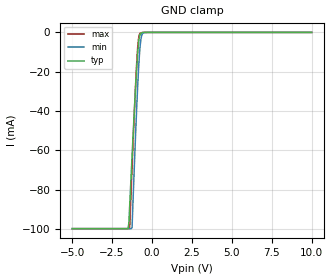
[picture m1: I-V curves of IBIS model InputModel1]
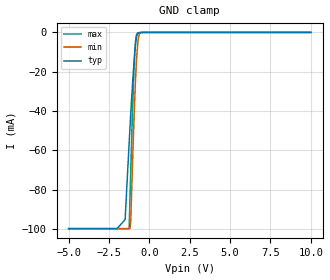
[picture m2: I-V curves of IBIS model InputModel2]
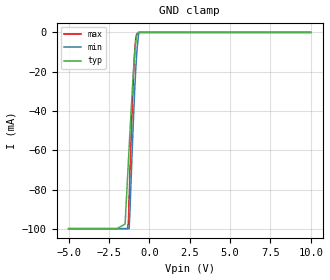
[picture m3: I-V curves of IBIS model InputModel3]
[IBIS Ver]   2.1
[File name]   e_002bl5.ibs   | e_= TSOP, f002bl= abbr chip name, 5= 5V Vcc
[File Rev]   2.00
[Date]   16-February-96
[Source]   File generated from lab measurements at Intel Corporation
[Notes]   Rev 2.00 All data was replaced by actual measurements
   performed in a lab.
[Disclaimer] INTEL DEVELOPER'S SOFTWARE LICENSE AGREEMENT
| BY USING THIS SOFTWARE, YOU ARE AGREEING TO BE BOUND
| BY THE TERMS OFTHIS AGREEMENT.  DO NOT USE THE SOFTWARE
| UNTIL YOU HAVE CAREFULLY READAND AGREED TO THE FOLLOWING
| TERMS AND CONDITIONS.  IF YOU DO NOT AGREETO THE TERMS
| OF THIS AGREEMENT, PROMPTLY RETURN THE SOFTWARE PACKAGE
| ANDANY ACCOMPANYING ITEMS.
| IF YOU USE THIS SOFTWARE, YOU WILL BE BOUND BY THE TERMS
| OF THIS AGREEMENT
| LICENSE: Intel Corporation ("Intel") grants you the non-exclusive right
| to use the enclosed software program ("Software").  You will not use,
| copy, modify, rent, sell or transfer the Software or any portion
| thereof, except as provided in this Agreement.
| System OEM Developers may:
| 1.   Copy the Software for support, backup or archival purposes;
| 2.   Install, use, or distribute Intel owned Software in object code
|   only;
| 3.   Modify and/or use Software source code that Intel directly makes
|   available to you as an OEM Developer;
| 4.   Install, use, modify, distribute, and/or make or have made
|   derivatives ("Derivatives") of Intel owned Software under the
|   terms and conditions in this Agreement, ONLY if you are a System
|   OEM Developer and NOT an end-user.
| RESTRICTIONS:
| YOU WILL NOT:
| 1.   Copy the Software, in whole or in part, except as provided for
|   in this Agreement;
| 2.   Decompile or reverse engineer any Software provided in object
|   code format;
| 3.   Distribute any Software or Derivative code to any end-users,
|   unless approved by Intel in a prior writing.
| TRANSFER: You may transfer the Software to another OEM
| Developer if thereceiving party agrees to the terms of this
| Agreement at the sole risk of any receiving party.
| OWNERSHIP AND COPYRIGHT OF SOFTWARE:
| Title to the Software and all copies thereof remain with Intel
| or its vendors.  The Software iscopyrighted and is protected by
| United States and international copyright laws.  You will not
| remove the copyright notice from the Software.  You agree to
| prevent any unauthorized copying of the Software.
| DERIVATIVE WORK: OEM Developers that make or have made
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[Copyright]   Copyright 1996, Intel Corporation, All Rights Reserved
[Component]   E28F002BL   | 40-lead TSOP package, 28F002BL
[Manufacturer]  Intel   | Boot Block (tm)
|   | operating in 5V Vcc range
[Package]
| The following values apply for the Alloy-42 leadframe.
|Variable   typ   min   max
R_pkg   135m   126m   144m
L_pkg   3.95nH   3.62nH   4.28nH
C_pkg   0.39pF   0.38pF   0.40pF
|***********************Pin Definition********************************
[Pin]   signal_name   model_name   R_pin   L_pin   C_pin
  1   A16   InputModel2
  2   A15   InputModel1
  3   A14   InputModel1
  4   A13   InputModel1
  5   A12   InputModel1
  6   A11   InputModel1
  7   A9   InputModel1
  8   A8   InputModel1
  9   WE#   InputModel5
 10   RP#   InputModel3
 11   VPP   POWER
 12   DU   InputModel6
 13   NC   InputModel1
 14   A7   InputModel1
 15   A6   InputModel1
 16   A5   InputModel1
 17   A4   InputModel1
 18   A3   InputModel1
 19   A2   InputModel1
 20   A1   InputModel1
 21   A0   InputModel2
 22   CE#   InputModel2
 23   GND   GND
 24   OE#   InputModel4
 25   DQ0   InputOutput
 26   DQ1   InputOutput
 27   DQ2   InputOutput
 28   DQ3   InputOutput
 29   NC   InputModel2
 30   VCC   POWER
 31   VCC   POWER
 32   DQ4   InputOutput
 33   DQ5   InputOutput
 34   DQ6   InputOutput
 35   DQ7   InputOutput
 36   A10   InputModel1
 37   NC   InputModel6
 38   NC   InputModel6
 39   GND   GND
 40   A17   InputModel1
|***********************Input Model 6******************************
[Model]   InputModel6
Model_type   Input
|   Model for  DU & NC pins, excluding Pin #13.
Vinl = 0.8V
Vinh = 2.0V
|Variable   Typ   Min   Max
C_comp   5.61p   NA   7.6p
[Voltage Range]   5.0V   4.5V   5.5V
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| Models and submodels in the file (7): InputModel1 (Input), InputModel2 (Input), InputModel3 (Input), InputModel4 (Input), InputModel5 (Input), InputModel6 (Input), InputOutput (I/O)
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|*********************Input Model 1************************************
[Model]   InputModel1
Model_type   Input
|   Model for A[15:1] A[17] & NC (pin 13).
Vinl = 0.8V
Vinh = 2.0V
|Variable   Typ   Min   Max
C_comp   5.61p   NA   7.6p
[Voltage Range]   5.0V   4.5V   5.5V
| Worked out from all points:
|   GND clamp passes 1 mA (typ) near -0.75 V on its own axis
[GND_clamp]
|Voltage  I(typ)   I(min)   I(max)
-5V       -99.84mA   -99.85mA   -99.85mA
-1.5V     -99.84mA   -99.85mA   -99.85mA
-1.45V    -97.1mA    -99.85mA   -99.85mA
-1.4V     -88.66mA   -99.85mA   -99.85mA
-1.25V    -63.24mA   -99.36mA   -69.05mA
-1.05V    -31.09mA   -56.35mA   -30.63mA
-950mV    -16.83mA   -36.7mA    -14.35mA
-850mV    -5.99mA    -19.86mA   -3.6mA
-750mV    -1.015mA   -7.435mA   -471.4uA
-650mV    -202.7uA   -1.654mA   -140.8uA
-500mV    -27.26uA   -101.4uA   -12.27uA
10V       0A         0A         0A
[Power_clamp]
| Input buffer circuits of this product do not intrinsically
| require a [Power_clamp] definition.  This zero current
| [Power_clamp] table is provided for the compatibility with
| some IBIS parsers.
|Voltage  I(typ)   I(min)   I(max)
-5V       0A         0A         0A
0V        0A         0A         0A
5V        0A         0A         0A
10V       0A         0A         0A
|*********************Input Model 2******************************
[Model]   InputModel2
Model_type   Input
|   Model for A[0], A[16] & CE# pins.
Vinl = 0.8V
Vinh = 2.0V
|Variable   Typ   Min   Max
C_comp   5.61p   NA   7.6p
[Voltage Range]   5.0V   4.5V   5.5V
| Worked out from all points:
|   GND clamp passes 1 mA (typ) near -0.75 V on its own axis
[GND_clamp]
|Voltage  I(typ)   I(min)   I(max)
-5V       -99.84mA   -99.85mA   -99.85mA
-2V       -99.84mA   -99.85mA   -99.85mA
-1.5V     -95.21mA   -99.85mA   -99.85mA
-1.25V    -55.95mA   -99.85mA   -99.68mA
-1.2V     -48.44mA   -99.85mA   -84.47mA
-1.15V    -41.14mA   -95.68mA   -69.64mA
-950mV    -15.15mA   -43.95mA   -18.45mA
-850mV    -5.666mA   -23.02mA   -4.089mA
-750mV    -1.032mA   -9.168mA   -475.6uA
-650mV    -207.5uA   -1.728mA   -133.8uA
-500mV    -28.64uA   -98.99uA   -10.29uA
10V       0A         0A         0A
[Power_clamp]
| Input buffer circuits of this product do not intrinsically
| require a [Power_clamp] definition.  This zero current
| [Power_clamp] table is provided for the compatibility with
| some IBIS parsers.
|Voltage  I(typ)   I(min)   I(max)
-5V       0A         0A         0A
0V        0A         0A         0A
5V        0A         0A         0A
10V       0A         0A         0A
|***********************Input Model 3******************************
[Model]   InputModel3
Model_type   Input
|   Model for RP# pin.
Vinl = 0.8V
Vinh = 2.0V
|Variable   Typ   Min   Max
C_comp   5.61p   NA   7.6p
[Voltage Range]   5.0V   4.5V   5.5V
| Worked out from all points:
|   GND clamp passes 1 mA (typ) near -0.75 V on its own axis
[GND_clamp]
|Voltage  I(typ)   I(min)   I(max)
-5V       -99.85mA   -99.85mA   -99.85mA
-2V       -99.85mA   -99.85mA   -99.85mA
-1.5V     -97.47mA   -99.85mA   -99.85mA
-1.35V    -73.75mA   -99.85mA   -99.85mA
-1.3V     -65.95mA   -99.85mA   -96.97mA
-1.25V    -58.19mA   -99.85mA   -83.97mA
-1.05V    -28.67mA   -57.7mA    -35.89mA
-950mV    -15.59mA   -37.45mA   -16.08mA
-850mV    -5.621mA   -20.13mA   -3.693mA
-750mV    -981uA     -7.476mA   -460uA
-650mV    0A         0A         0A
10V       0A         0A         0A
[Power_clamp]
| Input buffer circuits of this product do not intrinsically
| require a [Power_clamp] definition.  This zero current
| [Power_clamp] table is provided for the compatibility with
| some IBIS parsers.
|Voltage  I(typ)   I(min)   I(max)
-5V       0A         0A         0A
0V        0A         0A         0A
5V        0A         0A         0A
10V       0A         0A         0A
